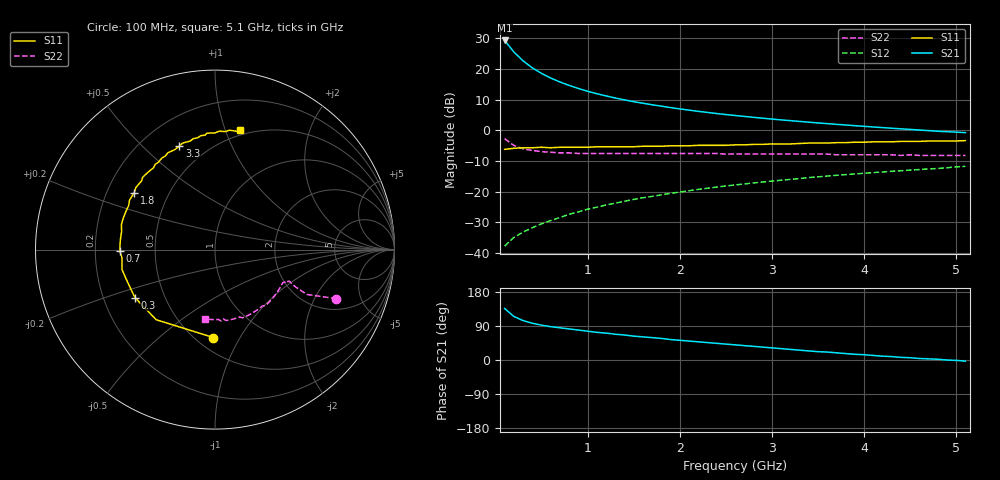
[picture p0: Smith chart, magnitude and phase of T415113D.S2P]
!AT-41511
!S-PARAMETERS at Vce=2.7V  Ic=25mA.  LAST UPDATED 01-25-95
# ghz s ma r 50
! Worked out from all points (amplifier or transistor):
!   51 points, 100 MHz to 5.1 GHz, reference 50 ohm
!   highest |S21| = 29.3 dB at 100 MHz (marker M1)
!   |S21| within 3 dB of that: start of sweep to 180.3 MHz
!   unconditionally stable (mu >= 1): 461.1 MHz to 4.008 GHz
!   at 900 MHz: K = 1.20, MAG = 17.4 dB, |S12| = -26.6 dB
!   at 2.6 GHz: K = 1.13, MAG = 9.1 dB, |S12| = -17.8 dB
!   at 5.1 GHz: K = 0.94, MSG = 5.5 dB, |S12| = -11.7 dB
!   lowest NFmin = 1.60 dB at 100 MHz
!   S11 on the Smith chart (normalised r, x): 100 MHz: 0.60, -0.78; 300 MHz: 0.34, -0.25; 700 MHz: 0.31, -0.01; 1.8 GHz: 0.32, +0.29; 3.3 GHz: 0.35, +0.65; 5.1 GHz: 0.46, +1.13
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0.1  0.49 -91.0  29.05 136.0  0.013 62.0  0.73 -22.0
0.2  0.51 -130.0  18.89 115.0  0.018 55.0  0.57 -26.0
0.3  0.52 -149.0  13.52 104.0  0.022 56.0  0.5 -25.0
0.4  0.52 -160.0  10.41 97.0  0.026 58.0  0.47 -24.0
0.5  0.53 -168.0  8.459 92.0  0.03 61.0  0.45 -23.0
0.6  0.52 -175.0  7.096 88.0  0.034 63.0  0.44 -24.0
0.7  0.53 -179.0  6.126 85.0  0.038 64.0  0.43 -24.0
0.8  0.53 176.0  5.384 82.0  0.043 65.0  0.43 -25.0
0.9  0.53 172.0  4.798 79.0  0.047 66.0  0.42 -26.0
1  0.53 169.0  4.33 76.0  0.052 67.0  0.42 -27.0
1.1  0.54 165.0  3.946 73.0  0.056 67.0  0.42 -28.0
1.3  0.54 159.0  3.361 68.0  0.065 67.0  0.42 -31.0
1.5  0.54 153.0  2.932 63.0  0.075 67.0  0.42 -34.0
1.8  0.55 145.0  2.473 57.0  0.089 66.0  0.42 -38.0
1.9  0.56 142.0  2.346 54.0  0.094 66.0  0.42 -40.0
2.2  0.57 135.0  2.038 48.0  0.109 65.0  0.42 -45.0
2.6  0.58 125.0  1.745 40.0  0.129 62.0  0.41 -51.0
3.3  0.61 109.0  1.396 26.0  0.164 57.0  0.41 -63.0
3.5  0.62 105.0  1.32 22.0  0.175 55.0  0.41 -66.0
3.9  0.64 97.0  1.189 15.0  0.195 52.0  0.4 -74.0
4.3  0.65 90.0  1.082 9.0  0.215 48.0  0.4 -81.0
5.1  0.68 78.0  0.917 -3.0  0.259 41.0  0.39 -98.0
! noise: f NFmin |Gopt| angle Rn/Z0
0.1  1.6  0.13  18  0.16
0.9  1.9  0.24  -162  0.13
1.8  2.3  0.4  -137  0.23
2.4  2.7  0.5  -122  0.35
